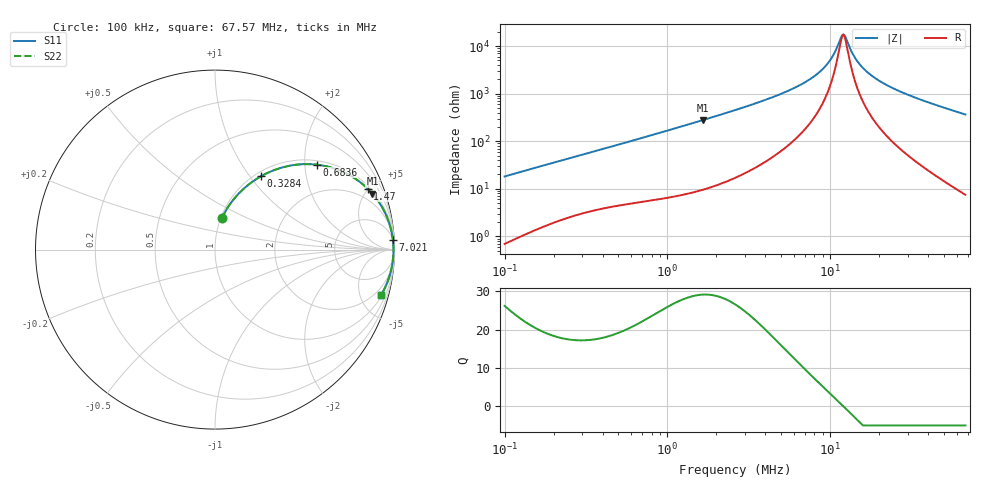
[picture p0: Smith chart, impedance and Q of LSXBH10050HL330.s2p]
! LSXBH10050HL330  S-PARAMETER MODEL  ( General Type )
! Model Generated by TAIYO YUDEN Corporation (http://www.ty-top.com)
! Version 3.0
! TAIYO YUDEN Control No. 180118NI43SB-FBB
! Copyright(c) 2007 TAIYO YUDEN CO.,LTD. All Rights Reserved.
! Product Description (link to TY-COMPAS)
! https://ds.yuden.co.jp/TYCOMPAS/or/detail?pn=LSXBH10050HL330M&u=M
! Products Name : Inductors
! Characteristics :
!  Inductance : 33 uH , SRF(min) : 8.2 MHz , DC Resistance(max) : 0.0858 Ohm
!  Rated Current : Saturation :2500 mA , Temp Rise : 2100 mA (40 degC)
!  Case Size : 10.0 x 9.8 / 0.394 x 0.386 [mm/inch] , Thickness : 5 / 0.197 [mm/inch]
!  (Conditions: Temperature = 25 degC , DC Bias Current/Voltage = 0A / 0V)
! External Node Assignments :
!  1  o---GGG---o  2
! GND o---------o GND
! Frequency Range : 0.1MHz  -  67.570357MHz  [ 402 STEP ]
# MHz S RI R 50
! Freq[MHz].  S11 Real  S11 Imag  S21 Real  S21 Imag  S12 Real  S12 Imag  S22 Real  S22 Imag
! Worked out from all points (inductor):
!   401 points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, 100 kHz to 67.57 MHz, reference 50 ohm
!   read as one part in series: L = 28.7 uH near 103.3 kHz
!   highest Q = 29.1 at 1.647 MHz (marker M1), where L = 26.8 uH
!   self-resonance near 12.02 MHz
!   S11 on the Smith chart (normalised r, x): 100 kHz: 1.01, +0.36; 328.4 kHz: 1.07, +1.13; 683.6 kHz: 1.10, +2.30; 1.47 MHz: 1.17, +4.94; 7.021 MHz: 5, +35; 67.57 MHz: 1.15, -7.29
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0.1  0.0381 0.1734  0.9619 -0.1734  0.9619 -0.1734  0.0381 0.1734
0.297841  0.2244 0.3891  0.7756 -0.3891  0.7756 -0.3891  0.2244 0.3891
0.328421  0.256 0.4084  0.744 -0.4084  0.744 -0.4084  0.256 0.4084
0.683562  0.5661 0.4733  0.4339 -0.4733  0.4339 -0.4733  0.5661 0.4733
0.887091  0.6814 0.4461  0.3186 -0.4461  0.3186 -0.4461  0.6814 0.4461
1.469855  0.8507 0.3395  0.1493 -0.3395  0.1493 -0.3395  0.8507 0.3395
1.647385  0.8769 0.3118  0.1231 -0.3118  0.1231 -0.3118  0.8769 0.3118
2.59943  0.9458 0.2083  0.0542 -0.2083  0.0542 -0.2083  0.9458 0.2083
4.74931  0.9824 0.1052  0.0176 -0.1052  0.0176 -0.1052  0.9824 0.1052
7.021274  0.9909 0.0561  0.00909 -0.0561  0.00909 -0.0561  0.9909 0.0561
7.742162  0.9921 0.0452  0.00791 -0.0452  0.00791 -0.0452  0.9921 0.0452
9.725316  0.9938 0.0213  0.00619 -0.0213  0.00619 -0.0213  0.9938 0.0213
10.55056  0.9941 0.0131  0.00588 -0.0131  0.00588 -0.0131  0.9941 0.0131
11.63381  0.9943 0.00333  0.00569 -0.00333  0.00569 -0.00333  0.9943 0.00333
12.01907  0.9943 7.96e-05  0.00567 -7.96e-05  0.00567 -7.96e-05  0.9943 7.96e-05
12.41708  0.9943 -0.00317  0.00567 0.00317  0.00567 0.00317  0.9943 -0.00317
14.14538  0.9941 -0.0162  0.0059 0.0162  0.0059 0.0162  0.9941 -0.0162
15.59772  0.9937 -0.0262  0.00631 0.0262  0.00631 0.0262  0.9937 -0.0262
18.35714  0.9925 -0.0433  0.00749 0.0433  0.00749 0.0433  0.9925 -0.0433
23.05932  0.9896 -0.0692  0.0104 0.0692  0.0104 0.0692  0.9896 -0.0692
36.38559  0.9766 -0.1319  0.0234 0.1319  0.0234 0.1319  0.9766 -0.1319
67.57036  0.9256 -0.2524  0.0744 0.2524  0.0744 0.2524  0.9256 -0.2524
